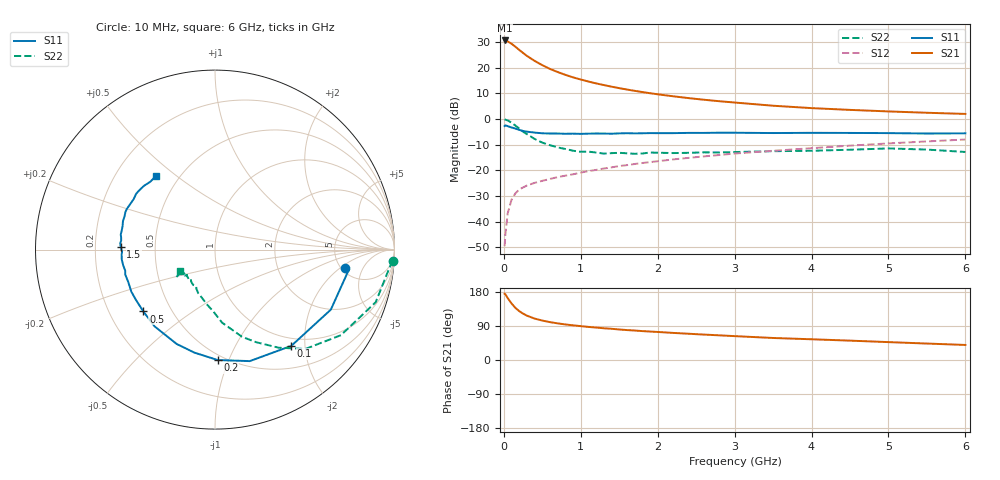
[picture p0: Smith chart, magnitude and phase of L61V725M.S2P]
!  INFINEON TECHNOLOGIES Small Signal Semiconductors
! BFR380L3 , Si-NPN RF-Transistor in TSLP-3-1
!  Vce=1.75 V,  Ic=25 mA
! Common Emitter S-Parameters:  07. March 2005
#  GHz  S  MA  R  50
! f  S11  S21  S12  S22
! GHz  Mag  Ang  Mag  Ang  Mag  Ang  Mag  Ang
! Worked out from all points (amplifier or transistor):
!   36 points, 10 MHz to 6 GHz, reference 50 ohm
!   highest |S21| = 30.7 dB at 10 MHz (marker M1)
!   |S21| within 3 dB of that: start of sweep to 172.4 MHz
!   unconditionally stable (mu >= 1): 1.873 GHz to 4.887 GHz
!   at 250 MHz: K = 0.38, MSG = 26.3 dB, |S12| = -26.7 dB
!   at 1.4 GHz: K = 0.96, MSG = 15.8 dB, |S12| = -18.9 dB
!   at 6 GHz: K = 0.98, MSG = 5.0 dB, |S12| = -8.0 dB
!   S11 on the Smith chart (normalised r, x): 10 MHz: 5.37, -2.39; 100 MHz: 0.86, -1.74; 200 MHz: 0.46, -0.91; 500 MHz: 0.35, -0.33; 1.5 GHz: 0.31, +0.01; 6 GHz: 0.37, +0.43
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0.01  0.7322 -8.1  34.24 174.8  0.0033 85.2  0.9914 -3.6
0.02  0.7546 -8.4  33.84 173.5  0.0056 85.0  0.9701 -7.5
0.05  0.7269 -27.4  32.84 163.4  0.0144 78.9  0.9422 -18.1
0.1  0.6844 -51.6  29.51 149.2  0.0267 67.7  0.8483 -34.2
0.15  0.6508 -72.7  25.86 137.6  0.0354 60.2  0.7483 -47.7
0.2  0.6155 -88.6  22.39 129.0  0.0422 56.7  0.6519 -57.0
0.25  0.5854 -101.3  19.55 122.4  0.0463 52.7  0.565 -66.0
0.3  0.5675 -112.1  17.11 117.0  0.0504 51.8  0.5083 -72.8
0.4  0.5442 -128.3  13.66 109.3  0.0568 50.3  0.4092 -84.4
0.5  0.5274 -139.2  11.28 104.1  0.0623 50.8  0.3468 -91.3
0.6  0.5222 -147.4  9.515 99.9  0.0678 51.8  0.3089 -98.3
0.8  0.516 -159.3  7.3 93.8  0.0785 55.1  0.2605 -111.0
0.9  0.519 -164.4  6.512 91.5  0.0835 56.2  0.2409 -115.6
1.1  0.5192 -170.5  5.398 87.3  0.0964 58.2  0.2314 -121.9
1.5  0.5254 178.5  4.015 80.5  0.1208 60.6  0.2195 -132.1
1.8  0.5277 172.4  3.369 76.3  0.1386 61.5  0.2124 -137.5
2.2  0.5311 165.8  2.786 71.5  0.1629 62.4  0.2168 -140.4
2.8  0.5415 157.0  2.232 65.1  0.1987 62.9  0.2229 -146.5
3.5  0.5333 148.3  1.821 58.1  0.2403 61.3  0.236 -145.6
4.5  0.5358 141.9  1.51 51.1  0.3027 60.0  0.2519 -145.2
5.5  0.5223 133.7  1.327 43.4  0.3659 56.4  0.2537 -145.2
6  0.5263 128.6  1.26 39.7  0.3988 54.3  0.2277 -148.2
